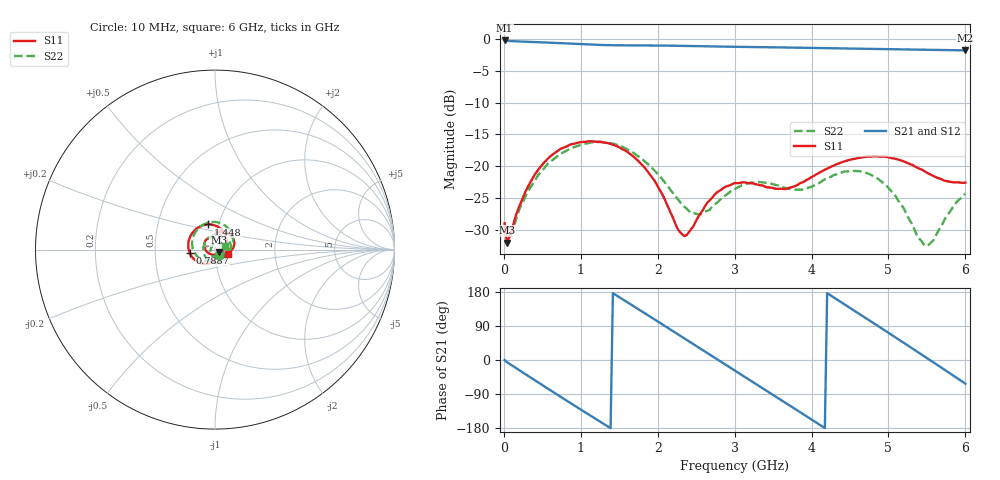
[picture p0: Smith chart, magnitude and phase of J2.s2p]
!Agilent Technologies,E8364B,MY43040528,A.07.50.67
!Agilent E8364B: A.07.50.67
!Date: Sunday, September 28, 2025 22:04:18
!Correction: S11(Full 2 Port(1,2))
!S21(Full 2 Port(1,2))
!S12(Full 2 Port(1,2))
!S22(Full 2 Port(1,2))
!S2P File: Measurements: S11, S21, S12, S22:
# Hz S  dB  R 50
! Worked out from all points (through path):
!   201 points, 10 MHz to 6 GHz, reference 50 ohm
!   highest |S21| = -0.27 dB at 10 MHz (marker M1); lowest = -1.8 dB at 6 GHz (marker M2)
!   group delay of S21, straight-line fit = 360 ps
!   lowest |S11| = -32.0 dB at 39.95 MHz (marker M3), VSWR 1.05, Z = 52.1 - j1.52 ohm
!   |S11| at or under -10 dB: start of sweep to end of sweep
!   |S22| runs from -32.5 to -16.2 dB; largest |S21 - S12| = 0.0074
!   S11 on the Smith chart (normalised r, x): 10 MHz: 1.04, -0.06; 788.7 MHz: 0.75, -0.03; 1.448 GHz: 0.89, +0.26; 6 GHz: 1.15, -0.05
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1e7  -28.94 -52.0  -0.27 -0.1  -0.30 0.2  -29.35 -54.9
3.995e7  -31.97 -35.4  -0.32 -5.6  -0.33 -5.1  -32.10 -37.3
4.293e8  -20.84 -119.0  -0.53 -57.0  -0.54 -56.9  -21.71 -132.3
7.887e8  -17.01 -171.7  -0.72 -103.6  -0.72 -103.6  -17.71 168.0
1.0283e9  -16.18 157.5  -0.86 -134.4  -0.86 -134.3  -16.55 132.0
1.4476e9  -16.77 104.8  -1.03 172.5  -1.02 172.6  -16.55 73.8
1.71715e9  -18.82 68.8  -1.05 138.2  -1.05 138.3  -18.19 38.0
2.01665e9  -23.52 21.9  -1.07 99.7  -1.07 99.8  -21.41 2.2
2.3461e9  -30.92 -80.0  -1.12 57.2  -1.12 57.3  -26.37 -19.2
2.55575e9  -27.41 -155.7  -1.17 30.1  -1.17 30.2  -27.56 -15.3
3.005e9  -22.62 134.2  -1.26 -27.8  -1.26 -27.7  -23.57 -40.2
3.27455e9  -22.83 110.2  -1.31 -62.6  -1.31 -62.5  -22.48 -75.6
3.51415e9  -23.49 99.6  -1.35 -93.7  -1.34 -93.6  -22.87 -115.9
3.75375e9  -23.24 97.1  -1.39 -124.9  -1.39 -124.8  -23.69 -166.7
4.0233e9  -21.55 90.5  -1.45 -160.1  -1.45 -160.0  -23.06 128.0
4.29285e9  -19.86 76.1  -1.51 164.7  -1.51 164.8  -21.37 71.9
4.59235e9  -18.75 56.2  -1.57 125.5  -1.58 125.6  -20.75 19.2
5.01165e9  -18.64 25.8  -1.65 70.2  -1.65 70.4  -23.55 -52.7
5.2812e9  -19.66 7.6  -1.69 34.4  -1.69 34.6  -28.56 -114.1
5.5208e9  -21.16 -3.8  -1.72 2.3  -1.72 2.5  -32.34 149.7
5.7604e9  -22.35 -10.0  -1.77 -30.0  -1.77 -29.8  -27.79 66.6
6e9  -22.57 -18.6  -1.82 -62.5  -1.82 -62.3  -24.32 18.5
